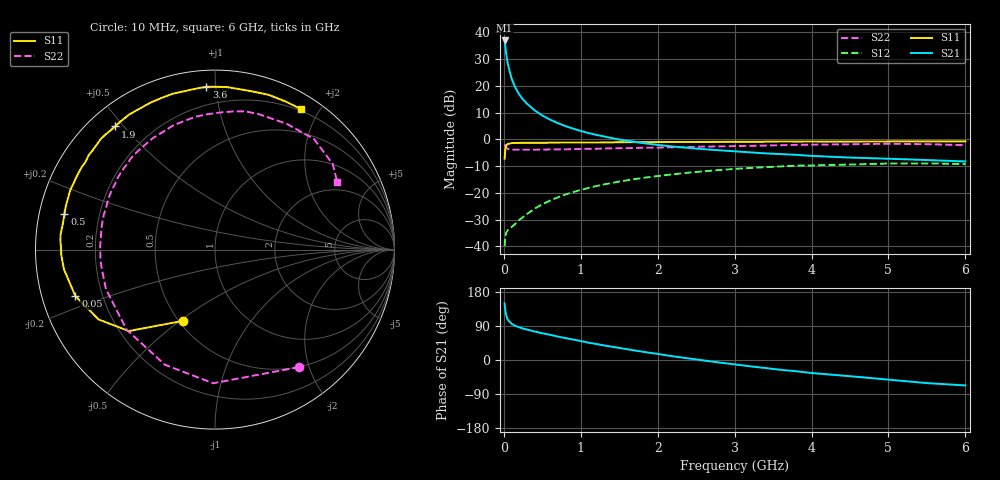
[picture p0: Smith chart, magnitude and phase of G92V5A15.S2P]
! SIEMENS Small Signal Semiconductors
! BFG235
! Si NPN RF Bipolar Junction Transistor in SOT223
! VCE = 2.5 V  IC = 150 mA
! Common Emitter S-Parameters:  July  1994
# GHz  S  MA  R  50
!  f  S11  S21  S12  S22
! GHz  MAG  ANG  MAG  ANG  MAG  ANG  MAG  ANG
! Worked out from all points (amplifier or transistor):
!   40 points, 10 MHz to 6 GHz, reference 50 ohm
!   highest |S21| = 36.9 dB at 10 MHz (marker M1)
!   |S21| within 3 dB of that: start of sweep to 22.29 MHz
!   unconditionally stable (mu >= 1): 430.1 MHz to 1.55 GHz
!   at 200 MHz: K = 0.82, MSG = 23.5 dB, |S12| = -30.1 dB
!   at 1.5 GHz: K = 1.01, MAG = 7.3 dB, |S12| = -15.8 dB
!   at 6 GHz: K = 0.92, MSG = 0.5 dB, |S12| = -9.2 dB
!   S11 on the Smith chart (normalised r, x): 10 MHz: 0.53, -0.51; 50 MHz: 0.10, -0.16; 500 MHz: 0.08, +0.12; 1.9 GHz: 0.08, +0.47; 3.6 GHz: 0.09, +0.94; 6 GHz: 0.18, +1.76
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0.01  0.4343 -114.0  70.2 149.3  0.0101 59.3  0.8055 -54.3
0.02  0.6605 -136.6  52.85 129.6  0.0153 45.1  0.7449 -90.8
0.03  0.7562 -149.0  40.41 118.1  0.0177 37.9  0.6995 -113.5
0.05  0.8198 -161.6  26.32 106.5  0.0201 32.0  0.6646 -137.9
0.1  0.8487 -172.6  13.75 95.5  0.023 36.0  0.646 -160.1
0.15  0.8567 -177.8  9.205 89.9  0.0264 43.0  0.6396 -169.3
0.2  0.858 179.3  6.884 86.3  0.0311 48.5  0.6412 -174.5
0.25  0.8631 176.6  5.541 83.0  0.0353 51.6  0.6393 -178.3
0.3  0.8647 174.5  4.629 80.4  0.0402 54.4  0.6402 178.5
0.4  0.8598 170.2  3.485 75.2  0.0507 56.9  0.6395 173.7
0.5  0.862 166.7  2.783 70.6  0.0612 57.9  0.6434 169.6
0.7  0.8683 160.1  2.015 61.9  0.0824 57.1  0.6494 162.3
0.9  0.8702 154.7  1.583 54.0  0.1033 54.1  0.655 156.0
1.1  0.8733 148.3  1.308 45.8  0.1237 50.5  0.6643 149.7
1.5  0.8809 138.5  0.991 31.8  0.1624 42.1  0.6814 138.0
1.9  0.8832 129.0  0.818 18.9  0.1976 33.1  0.6976 127.0
2.2  0.8916 122.5  0.733 9.7  0.2222 26.3  0.7112 119.1
3.2  0.8988 101.2  0.571 -16.6  0.2913 3.0  0.7552 93.2
3.6  0.9084 93.0  0.53 -26.0  0.3118 -6.8  0.7767 82.4
4.5  0.9051 77.6  0.456 -42.8  0.3382 -26.2  0.8068 60.3
5.5  0.9141 64.6  0.41 -61.0  0.3552 -47.6  0.8108 36.0
6  0.9174 58.7  0.386 -67.1  0.3455 -55.7  0.7786 29.0
